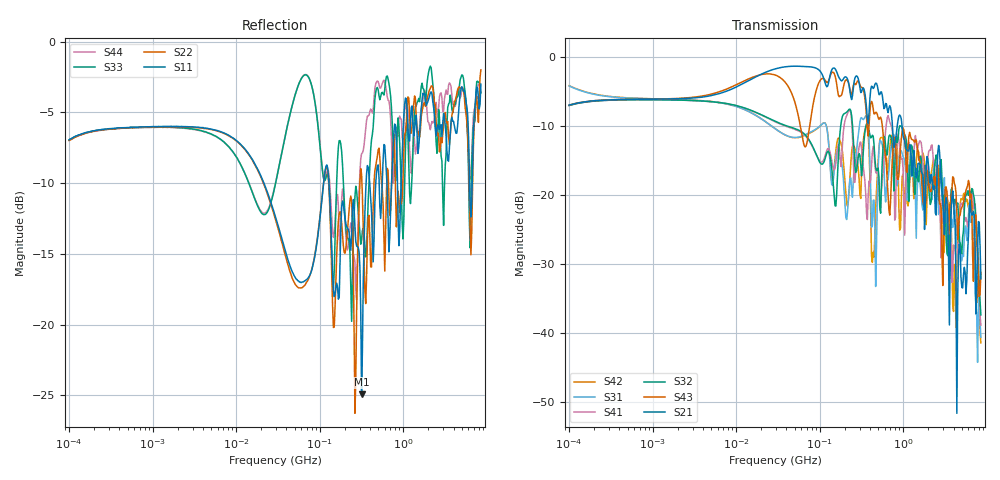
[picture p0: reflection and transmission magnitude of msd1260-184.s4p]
# MHz S MA R 50
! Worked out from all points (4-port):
!   498 points, 100 kHz to 8.5 GHz, reference 50 ohm
!   strongest paths, dB at 100 kHz, 1.698 MHz, 29.49 MHz, 500.7 MHz, 8.5 GHz:
!     S21: -7.0, -6.1, -1.8, -4.8, -32.2
!     S43: -7.0, -6.1, -2.7, -8.8, -31.3
!     S32: -7.1, -6.3, -9.4, -16.1, -37.4
!     S41: -7.1, -6.3, -9.4, -16.9, -38.9
!     S31: -4.2, -6.2, -10.4, -16.3, -40.6
!     S42: -4.2, -6.2, -10.4, -15.2, -41.5
!   lowest |S11| = -24.9 dB at 317.1 MHz (marker M1), VSWR 1.12, Z = 55.2 - j2.94 ohm
!   |S11| at or under -10 dB: 21.5 MHz to 111.4 MHz (89.89 MHz wide, 135 % of centre); 128.9 MHz to 359.3 MHz (230.3 MHz wide, 94.4 % of centre); 6.227 GHz to 6.69 GHz (462.7 MHz wide, 7.16 % of centre)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
0.1  0.4499 24.2  0.446 24.8  0.6141 -18.1  0.443 -155.9
     0.446 24.8  0.4477 24.3  0.4436 -155.8  0.6164 -18.0
     0.6141 -18.1  0.4436 -155.8  0.4489 24.3  0.4457 24.7
     0.443 -155.9  0.6164 -18.0  0.4457 24.7  0.4485 24.3
317.0858  0.05658 -28.0  0.5566 -64.9  0.362 10.8  0.2158 -38.3
          0.5566 -64.9  0.34 -28.5  0.1373 -2.6  0.1466 35.0
          0.362 10.8  0.1373 -2.6  0.1997 -17.0  0.5996 -81.1
          0.2158 -38.3  0.1466 35.0  0.5996 -81.1  0.4019 12.7
601.0223  0.4301 -62.8  0.428 -106.8  0.1075 -73.8  0.2435 -0.9
          0.428 -106.8  0.1545 -55.9  0.2606 -44.4  0.2026 -44.4
          0.1075 -73.8  0.2606 -44.4  0.6793 -62.2  0.2076 -163.7
          0.2435 -0.9  0.2026 -44.4  0.2076 -163.7  0.7216 -77.5
2159.325  0.6654 -178.4  0.1403 102.6  0.09544 131.1  0.2264 130.7
          0.1403 102.6  0.6972 -176.8  0.08956 146.6  0.1432 138.4
          0.09544 131.1  0.08956 146.6  0.8085 171.1  0.1056 -33.1
          0.2264 130.7  0.1432 138.4  0.1056 -33.1  0.5084 -171.8
3568.796  0.4212 16.8  0.01139 -124.4  0.02587 -115.6  0.06835 -10.0
          0.01139 -124.4  0.4327 4.1  0.02452 -103.7  0.076 -8.4
          0.02587 -115.6  0.02452 -103.7  0.6095 12.4  0.07564 33.9
          0.06835 -10.0  0.076 -8.4  0.07564 33.9  0.7157 4.3
5898.28  0.5538 -140.3  0.03879 113.7  0.04659 159.5  0.05867 160.7
         0.03879 113.7  0.4656 -142.2  0.1067 157.5  0.0865 128.4
         0.04659 159.5  0.1067 157.5  0.4619 -155.5  0.1165 62.6
         0.05867 160.7  0.0865 128.4  0.1165 62.6  0.5188 -144.9
8500  0.708 -39.3  0.0246 -131.8  0.00929 -63.7  0.01139 -123.7
      0.0246 -131.8  0.7951 -44.7  0.01348 -123.2  0.008447 -102.1
      0.00929 -63.7  0.01348 -123.2  0.6593 -56.4  0.02738 15.4
      0.01139 -123.7  0.008447 -102.1  0.02738 15.4  0.661 -57.4
